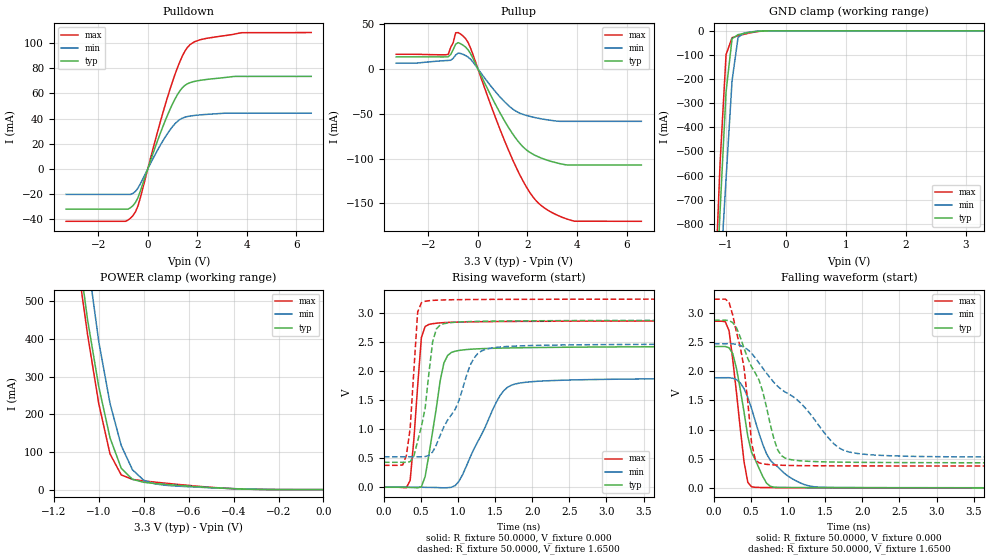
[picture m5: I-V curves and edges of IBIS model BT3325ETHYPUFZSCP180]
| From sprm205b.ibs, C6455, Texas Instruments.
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|   Model BT3325ETHYPUFZSCP180
[Model]   BT3325ETHYPUFZSCP180
Model_type   I/O
Polarity   Non-Inverting
Enable   Active-Low
Vinl =   0.8000V
Vinh =   2.0000V
Vmeas =   1.5000V
Cref =  20.0000pF
Rref =  25.0000
Vref =   1.5000V
C_comp   2.0747pF   2.0118pF   2.1577pF
[Temperature Range]   25.0000   0.1250k   -40.0000
[Pullup Reference]   3.3000V   3.0000V   3.6000V
[Pulldown Reference]   0.000V   0.000V   0.000V
[POWER Clamp Reference]   3.3000V   3.0000V   3.6000V
[GND Clamp Reference]   0.000V   0.000V   0.000V
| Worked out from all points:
|   slope of the pulldown table from 0 to 0.495 V, typ, clamps not added: 17.8 ohm
|   slope of the pullup table from 0 to 0.495 V, typ, clamps not added: 17.6 ohm
|   GND clamp passes 1 mA (typ) near -0.42 V on its own axis
|   POWER clamp passes 1 mA (typ) near -0.32 V on its own axis
|   rising waveform, R_fixture 50.0000, V_fixture 0.000: 20-80 % time 179ps typ, 416ps min, 102ps max; typ from 0 V to 2.42 V
|   rising waveform, R_fixture 50.0000, V_fixture 1.6500: 20-80 % time 166ps typ, 391ps min, 90.3ps max; typ from 0.43 V to 2.87 V
|   falling waveform, R_fixture 50.0000, V_fixture 0.000: 20-80 % time 236ps typ, 374ps min, 150ps max; typ from 2.42 V to 0 V
|   falling waveform, R_fixture 50.0000, V_fixture 1.6500: 20-80 % time 384ps typ, 866ps min, 190ps max; typ from 2.87 V to 0.429 V
[Pulldown]
| voltage   I(typ)   I(min)   I(max)
-3.3V     -32.13mA   -20.39mA   -41.8mA
-800mV    -32.13mA   NA         -40.84mA
-600mV    -29.35mA   -19.57mA   -37.3mA
-400mV    -23.06mA   -15.47mA   -29.75mA
400mV     22.69mA    15.1mA     29.91mA
900mV     47.48mA    31.04mA    63.55mA
1.2V      59.18mA    37.83mA    80.66mA
1.4V      64.67mA    40.4mA     90mA
1.7V      68.56mA    41.99mA    98.77mA
2.2V      70.71mA    43.08mA    103.2mA
3.5V      73.58mA    NA         107.3mA
6.6V      73.58mA    44.26mA    108.5mA
[Pullup]
| voltage   I(typ)   I(min)   I(max)
-3.3V     13.33mA    6.339mA    16.28mA
-1.2V     13.39mA    9.386mA    16.1mA
-1V       21.42mA    11.73mA    29.1mA
-900mV    27.5mA     15.41mA    40.23mA
-700mV    28.05mA    17.16mA    38.77mA
-300mV    17.07mA    10.77mA    23.36mA
700mV     -39.18mA   -25.19mA   -53.66mA
1.4V      -72.33mA   -44.64mA   -101.1mA
1.9V      -88.97mA   -51.43mA   -128.9mA
2.4V      -97.57mA   -54.84mA   -148.4mA
3.6V      -107.1mA   NA         -167.4mA
6.6V      -107.2mA   -58.47mA   -169.9mA
[GND_clamp]
| voltage   I(typ)   I(min)   I(max)
-3.3V     -15.89A    -14.36A    -17.09A
-1.2V     -1.272A    -1.463A    -1.17A
-1.1V     -747.6mA   -1.03A     -548.7mA
-1V       -252.9mA   -612.9mA   -98.87mA
-900mV    -32.78mA   -207mA     -28.39mA
-800mV    -15.81mA   -27.43mA   -20.51mA
-700mV    -10.59mA   -9.104mA   -14.4mA
-400mV    -643.1uA   -603.4uA   -1.056mA
3.3V      40.62nA    12.96uA    313nA
[POWER_clamp]
| voltage   I(typ)   I(min)   I(max)
-3.3V     13.85A     12.5A      14.97A
-1.1V     674.7mA    860.4mA    626.3mA
-1.05V    451.9mA    613.5mA    412.5mA
-1V       273.5mA    392.8mA    228.3mA
-950mV    137.6mA    229.1mA    94.87mA
-900mV    56.69mA    117mA      39.04mA
-850mV    27.31mA    52.64mA    27.23mA
-800mV    19.41mA    24.91mA    23.17mA
-750mV    16.13mA    15.16mA    19.95mA
-600mV    9.271mA    7.614mA    11.13mA
-350mV    1.4mA      1.652mA    1.221mA
0V        125.5nA    253.7nA    383.9nA
[Ramp]
| variable   typ   min   max
dV/dt_r   1.4534/0.1776n   1.1261/0.4115n   1.7179/0.1008n
dV/dt_f   1.4430/0.2676n   1.1285/0.5804n   1.6968/0.1551n
R_load = 50.0000
[Rising Waveform]
R_fixture = 50.0000
V_fixture = 0.000
V_fixture_min = 0.000
V_fixture_max = 0.000
| time   V(typ)   V(min)   V(max)
0s        33.52uV    39.09uV    47.3uV
303ps     -715.4uV   38.21uV    -7.114mV
353.5ps   -4.293mV   50.58uV    119.8mV
505.1ps   8.308mV    -308.2uV   2.579V
606.1ps   558.6mV    -3.172mV   2.802V
808.1ps   2.138V     -9.635mV   2.834V
959.6ps   2.342V     27.88mV    2.841V
1.515ns   2.393V     1.465V     2.852V
1.717ns   2.399V     1.756V     2.854V
5ns       2.422V     1.877V     2.863V
[Rising Waveform]
R_fixture = 50.0000
V_fixture = 1.6500
V_fixture_min = 1.5000
V_fixture_max = 1.8000
| time   V(typ)   V(min)   V(max)
0s        429.6mV    524.6mV    377.1mV
303ps     429.2mV    524.8mV    548.9mV
353.5ps   441.2mV    524.8mV    1.015V
454.5ps   793.7mV    524.7mV    3.018V
505.1ps   1.046V     524.7mV    3.175V
656.6ps   2.506V     607.6mV    3.216V
808.1ps   2.816V     1.04V      3.225V
1.212ns   2.854V     2.22V      3.232V
1.364ns   2.858V     2.371V     3.233V
5ns       2.874V     2.465V     3.238V
[Falling Waveform]
R_fixture = 50.0000
V_fixture = 0.000
V_fixture_min = 0.000
V_fixture_max = 0.000
| time   V(typ)   V(min)   V(max)
0s        2.424V     1.889V     2.858V
151.5ps   2.425V     1.889V     2.85V
202ps     2.402V     1.889V     2.695V
303ps     2.044V     1.853V     1.622V
404ps     1.3V       1.702V     448.5mV
454.5ps   886.6mV    1.553V     96.52mV
505.1ps   609.5mV    1.363V     18.58mV
757.6ps   26.86mV    474mV      4.556mV
1.263ns   4.668mV    39.01mV    1.273mV
5ns       246.7uV    1.436mV    33.1uV
[Falling Waveform]
R_fixture = 50.0000
V_fixture = 1.6500
V_fixture_min = 1.5000
V_fixture_max = 1.8000
| time   V(typ)   V(min)   V(max)
0s        2.874V     2.472V     3.236V
202ps     2.869V     2.473V     3.182V
252.5ps   2.832V     2.47V      2.959V
404ps     2.397V     2.412V     2.06V
505.1ps   2.078V     2.31V      775.7mV
606.1ps   1.849V     2.14V      429mV
858.6ps   649.7mV    1.741V     390.4mV
1.01ns    490.5mV    1.607V     384.7mV
1.818ns   439.2mV    616.2mV    376.7mV
5ns       428.6mV    524.5mV    374.2mV
